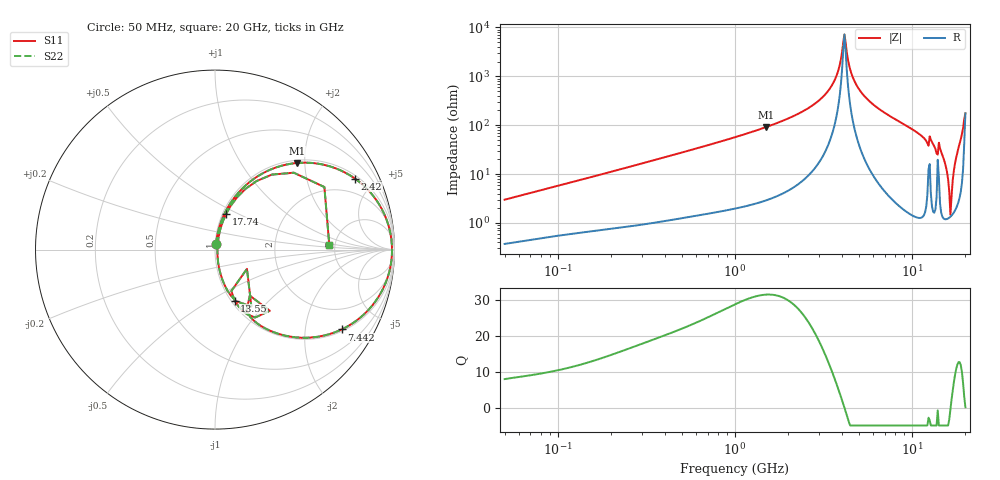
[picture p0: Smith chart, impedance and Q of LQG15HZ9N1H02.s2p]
!Murata Part Number: LQG15HZ9N1H02
!These Parameters are Measured in Series Mode Connection
!  o--[Z]--o
!Port1  Port2
!  o-------o
!Freq. Start=50[MHz] Stop=20[GHz], 401[Steps]
# Hz S RI R 50
!Freq.(Hz) S11(Real) S11(Imag) S21(Real) S21(Imag) S12(Real) S12(Imag) S22(Real) S22(Imag)
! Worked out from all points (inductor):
!   401 points, 50 MHz to 20 GHz, reference 50 ohm
!   read as one part in series: L = 9.31 nH near 51.52 MHz
!   highest Q = 31.6 at 1.498 GHz (marker M1), where L = 9.71 nH
!   self-resonance near 4.088 GHz
!   S11 on the Smith chart (normalised r, x): 50 MHz: 1.01, +0.06; 2.42 GHz: 1.15, +3.85; 7.442 GHz: 1.07, -3.12; 13.55 GHz: 1.04, -0.65; 17.74 GHz: 1.04, +0.43; 20 GHz: 4.49, +0.36
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5e7  0.00457 0.0294  0.9954 -0.0294  0.9954 -0.0294  0.00457 0.0294
1.364002e8  0.0121 0.0754  0.9879 -0.0754  0.9879 -0.0754  0.0121 0.0754
3.721004e8  0.0494 0.1927  0.9506 -0.1927  0.9506 -0.1927  0.0494 0.1927
1e9  0.2511 0.4167  0.7489 -0.4167  0.7489 -0.4167  0.2511 0.4167
1.498439e9  0.4571 0.4826  0.5429 -0.4826  0.5429 -0.4826  0.4571 0.4826
2.419936e9  0.7792 0.3961  0.2208 -0.3961  0.2208 -0.3961  0.7792 0.3961
2.728004e9  0.8526 0.3326  0.1474 -0.3326  0.1474 -0.3326  0.8526 0.3326
3.572216e9  0.967 0.1332  0.033 -0.1332  0.033 -0.1332  0.967 0.1332
4.149438e9  0.9863 -0.000172  0.0137 0.000172  0.0137 0.000172  0.9863 -0.000172
4.539627e9  0.9797 -0.0826  0.0203 0.0826  0.0203 0.0826  0.9797 -0.0826
4.966507e9  0.959 -0.1638  0.041 0.1638  0.041 0.1638  0.959 -0.1638
7.442007e9  0.705 -0.4451  0.295 0.4451  0.295 0.4451  0.705 -0.4451
1.034674e10  0.3716 -0.4745  0.6284 0.4745  0.6284 0.4745  0.3716 -0.4745
1.354865e10  0.1089 -0.2837  0.8911 0.2837  0.8911 0.2837  0.1089 -0.2837
1.460232e10  0.0869 -0.2546  0.9131 0.2546  0.9131 0.2546  0.0869 -0.2546
1.550395e10  0.0313 -0.1376  0.9687 0.1376  0.9687 0.1376  0.0313 -0.1376
1.597544e10  0.0179 -0.0748  0.9821 0.0748  0.9821 0.0748  0.0179 -0.0748
1.646126e10  0.0132 -0.00573  0.9868 0.00573  0.9868 0.00573  0.0132 -0.00573
1.696185e10  0.02 0.0706  0.98 -0.0706  0.98 -0.0706  0.02 0.0706
1.774144e10  0.0619 0.199  0.9381 -0.199  0.9381 -0.199  0.0619 0.199
1.912117e10  0.3172 0.4179  0.6828 -0.4179  0.6828 -0.4179  0.3172 0.4179
2e10  0.637 0.0237  0.363 -0.0237  0.363 -0.0237  0.637 0.0237
